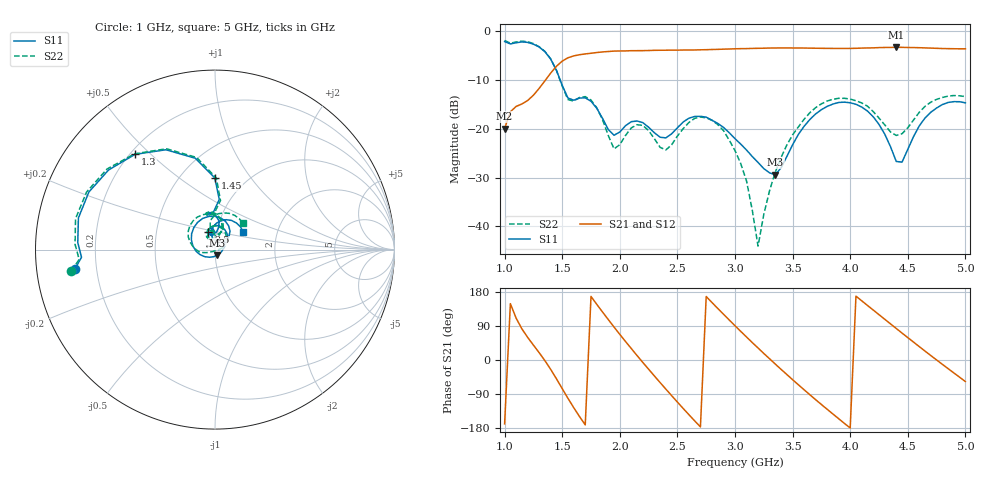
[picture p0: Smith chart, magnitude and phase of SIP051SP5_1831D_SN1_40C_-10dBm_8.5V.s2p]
# GHz  S  dB  R  50
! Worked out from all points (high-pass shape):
!   81 points, 1 GHz to 5 GHz, reference 50 ohm
!   highest |S21| = -3.25 dB at 4.4 GHz (marker M1); lowest = -19.9 dB at 1 GHz (marker M2)
!   |S21| within 3 dB of the highest: 1.492 GHz to end of sweep
!   lowest |S11| = -29.4 dB at 3.35 GHz (marker M3), VSWR 1.07, Z = 51.2 - j3.2 ohm
!   |S11| at or under -10 dB: 1.483 GHz to end of sweep
!   |S22| runs from -44.0 to -1.8 dB; largest |S21 - S12| = 0.0026
!   S11 on the Smith chart (normalised r, x): 1 GHz: 0.12, -0.07; 1.3 GHz: 0.22, +0.45; 1.45 GHz: 0.72, +0.69; 2.5 GHz: 0.91, +0.18; 5 GHz: 1.34, +0.28
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1  -2.07 -172.1  -19.92 -168.6  -19.89 -168.9  -1.85 -171.6
1.3  -3.19 130.0  -11.68 19.3  -11.69 19.4  -3.14 130.0
1.45  -7.98 90.2  -7.14 -49.6  -7.13 -49.5  -7.98 88.9
1.55  -13.66 92.6  -5.40 -101.2  -5.39 -101.2  -13.99 91.7
1.7  -13.62 97.6  -4.61 -171.1  -4.62 -171.2  -13.37 96.7
1.8  -15.76 82.4  -4.33 146.9  -4.33 147.0  -15.65 77.5
1.95  -21.29 98.7  -4.03 86.9  -4.04 86.9  -24.09 93.1
2.15  -18.37 102.5  -3.94 11.6  -3.94 11.6  -19.14 105.5
2.35  -21.70 96.9  -3.86 -59.5  -3.87 -59.6  -23.77 94.4
2.5  -19.75 110.7  -3.84 -111.1  -3.83 -111.1  -21.46 123.7
2.75  -17.58 71.9  -3.74 167.5  -3.74 167.4  -17.71 80.6
3  -21.99 33.8  -3.56 90.4  -3.56 90.4  -24.43 27.6
3.1  -24.33 21.3  -3.52 60.7  -3.51 60.6  -30.66 7.0
3.2  -26.87 3.0  -3.46 31.7  -3.45 31.7  -44.05 -70.7
3.35  -29.41 -67.3  -3.39 -10.8  -3.40 -10.7  -28.85 -154.5
3.55  -21.13 -161.3  -3.39 -65.4  -3.39 -65.4  -19.58 -179.5
3.7  -16.92 157.5  -3.44 -104.7  -3.45 -104.7  -15.63 154.3
4  -14.63 89.8  -3.48 -179.4  -3.48 -179.6  -13.86 100.6
4.35  -23.64 40.7  -3.28 95.4  -3.28 95.4  -20.61 74.0
4.4  -26.67 55.5  -3.25 83.2  -3.25 83.2  -21.33 84.1
4.7  -16.57 86.5  -3.42 11.7  -3.41 11.8  -14.50 91.4
5  -14.65 32.7  -3.56 -56.9  -3.56 -57.0  -13.36 42.9
